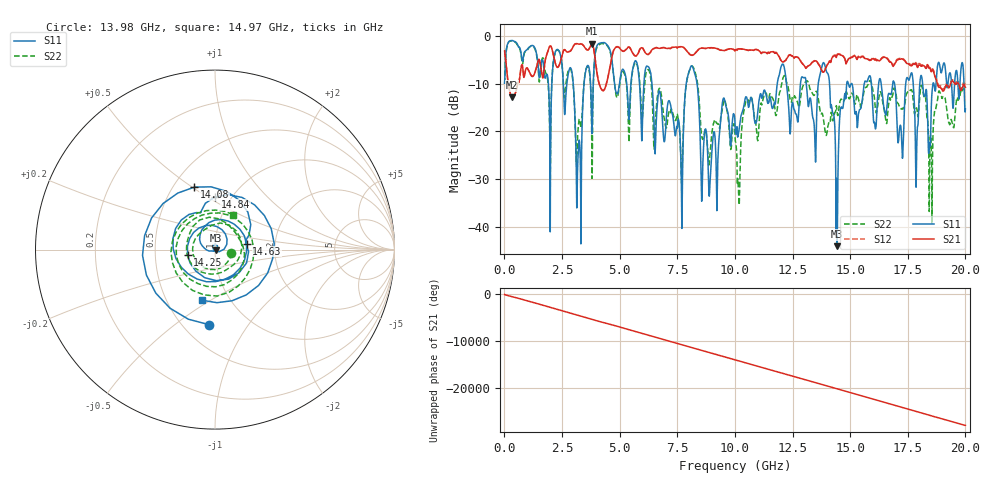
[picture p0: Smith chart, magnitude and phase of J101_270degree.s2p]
!Keysight Technologies,N5222A,MY51421036,A.10.65.16
!Date: Friday, March 31, 2023 14:51:25
!Correction: S11(Full 2 Port(1,2))
!S21(Full 2 Port(1,2))
!S12(Full 2 Port(1,2))
!S22(Full 2 Port(1,2))
!S2P File: Measurements: S11, S21, S12, S22:
# Hz S  dB  R 50
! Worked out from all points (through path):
!   2000 points, 10 MHz to 20 GHz, reference 50 ohm
!   highest |S21| = -1.60 dB at 3.8 GHz (marker M1); lowest = -12.9 dB at 330 MHz (marker M2)
!   group delay of S21, straight-line fit = 3.9 ns
!   lowest |S11| = -44.1 dB at 14.44 GHz (marker M3), VSWR 1.01, Z = 50.5 - j0.305 ohm
!   |S11| at or under -10 dB: 6.401 GHz to 7.889 GHz (1.488 GHz wide, 20.8 % of centre); 8.359 GHz to 11.84 GHz (3.479 GHz wide, 34.5 % of centre); 14.11 GHz to 14.85 GHz (745.1 MHz wide, 5.15 % of centre)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
!   |S22| runs from -39.5 to -1.0 dB; largest |S21 - S12| = 0.02
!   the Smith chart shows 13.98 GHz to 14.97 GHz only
!   S11 on the Smith chart (normalised r, x): 13.98 GHz: 0.66, -0.68; 14.08 GHz: 0.63, +0.51; 14.25 GHz: 0.73, -0.04; 14.63 GHz: 1.42, +0.10; 14.84 GHz: 0.84, +0.54; 14.97 GHz: 0.75, -0.46
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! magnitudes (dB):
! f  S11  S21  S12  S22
! 10 MHz  -9.9  -3.1  -3.1  -10.0
! 330 MHz  -0.9  -12.9  -12.9  -1.0
! 1.97 GHz  -20.2  -2.2  -2.1  -21.9
! 2.35 GHz  -3.0  -6.4  -6.4  -3.0
! 3.35 GHz  -24.4  -1.7  -1.6  -18.3
! 3.8 GHz  -20.5  -1.6  -1.5  -29.9
! 4.23 GHz  -1.4  -11.3  -11.3  -1.6
! 6.68 GHz  -12.1  -2.5  -2.5  -11.5
! 8.91 GHz  -31.6  -2.5  -2.5  -25.4
! 10.01 GHz  -19.1  -3.1  -3.1  -21.4
! 13.34 GHz  -15.5  -5.6  -5.6  -11.8
! 13.98 GHz  -7.5  -6.3  -6.2  -20.7
! 14.08 GHz  -8.7  -5.5  -5.4  -18.1
! 14.25 GHz  -16.2  -4.3  -4.3  -17.8
! 14.44 GHz  -44.1  -3.9  -3.8  -16.2
! 14.63 GHz  -14.9  -4.0  -4.0  -13.3
! 14.84 GHz  -10.7  -5.6  -5.6  -11.7
! 14.97 GHz  -10.7  -4.7  -4.6  -13.2
! 16.67 GHz  -12.0  -5.2  -5.0  -14.3
! 18.15 GHz  -10.2  -6.2  -6.0  -11.4
! 18.5 GHz  -19.1  -7.4  -7.1  -21.0
! 20 GHz  -15.3  -10.8  -10.4  -10.7
